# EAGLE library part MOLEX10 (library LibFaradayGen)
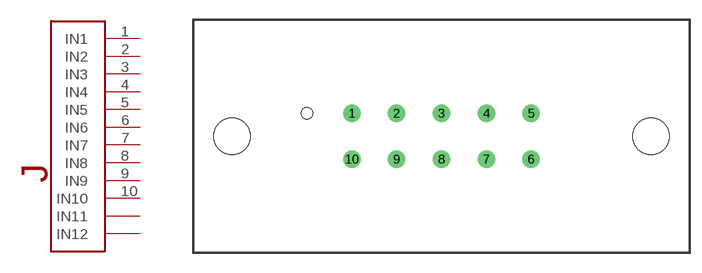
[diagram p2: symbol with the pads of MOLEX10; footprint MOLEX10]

Designator prefix J

## MOLEX10  [MOLEX10]
1  IN1  pas
2  IN2  pas
3  IN3  pas
4  IN4  pas
5  IN5  pas
6  IN6  pas
7  IN7  pas
8  IN8  pas
9  IN9  pas
10  IN10  pas

## Footprint MOLEX10 (pad centres in mm)
drill 1.52: 1 -11.68,2.995; 2 -5.84,2.995; 3 0,2.995; 4 5.84,2.995; 5 11.68,2.995; 6 11.68,-2.995; 7 5.84,-2.995; 8 0,-2.995; 9 -5.84,-2.995; 10 -11.68,-2.995
hole 1.52 at -17.52,2.995
hole 4.78 at -27.29,0
hole 4.78 at 27.29,0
